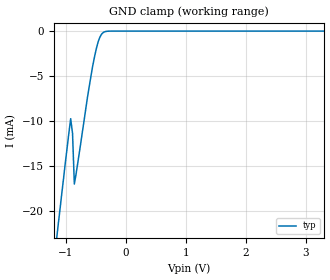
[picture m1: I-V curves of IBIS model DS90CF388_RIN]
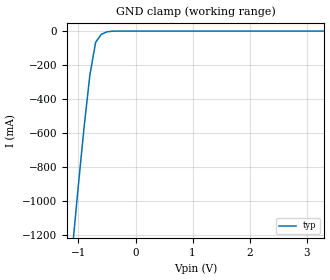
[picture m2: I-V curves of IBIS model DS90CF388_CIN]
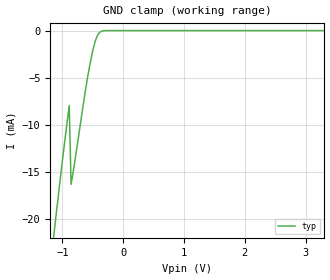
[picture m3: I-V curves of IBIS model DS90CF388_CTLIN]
|   National Semiconductor Corporation
|   Interface Products Group
|   IBIS Model of DS90CF388
|   100L TQFP Package
[IBIS Ver]   2.1
[File name]   90cf388.ibs
[File Rev]   1.0
[Date]   8/04/98
[Source]   File originated at National Semiconductor Corporation.
   Interface Group/Analog Division. All data based on
   measurements. CLKin and CLKout based on HSPICE sim.
[Notes]   File created/verfied by SBH.
[Disclaimer]
(C) Copyright National Semiconductor Corporation 1994
   All rights reserved
   National Semiconductor Corporation hereby grants
the user of this IBIS model a non-exclusive, nontransferable
license to use this IBIS model under the following terms.
Before using this IBIS model, the user should read this
license.  If the user does not accept these terms,  the
IBIS model should be returned to National within 30 days.
   The user is granted this license only to use the
IBIS model and is not granted rights to sell, load, rent,
lease or license the IBIS model in whole or in part, or in
modified form to anyone other than user. User may modify
the IBIS model to suit its specific applications but rights
to derivative works and such modifications shall belong to
National.
   This IBIS model is provided on an "AS IS" basis and
National makes absolutely no warranty with respect to the
information contained herein.NATIONAL DISCLAIMS AND CUSTOMER
WAIVES ALL WARRANTIES, EXPRESS OR IMPLIED, INCLUDING
WARRANTIES OF MERCHANTABILITY OR FITNESS FOR A PARTICULAR
PURPOSE. The entire risk as to quality and performance is
with the Customer. ACCORDINGLY, IN NO EVENT SHALL THE
COMPANY BE LIABLE FOR ANY DAMAGES, WHETHER IN CONTRACT OR
TORT,INCLUDING ANY LOST PROFITS OR OTHER INCIDENTAL,
CONSEQUENTIAL, EXEMPLARY, OR PUNITIVE DAMAGES ARISING OUT
OF THE USE OR APPLICATION OF THE IBIS model provided in
this package.Further, National reserves the right to make
changes without notice to any product herein to improve
reliability, function, or design. National does not convey
any license under patent rights or any other intellectual
property rights, including those of third parties.
   National is not obligated to provide maintenance or support
for the licensed IBIS model.
Contact National at ATTN:INTERFACE APPLICATIONS/IBIS MODELS.
2900 Semiconductor Drive, M/S A2595, Santa Clara, CA 95052-8090
[Copyright]   Copyright 1994, National Semiconductor, All Rights Reserved
[Component]   DS90CF388VJD
[Manufacturer]  National Semiconductor Corp
[Package]
|   typ   min   max
R_pkg   50.0m   NA   NA
L_pkg   2.52nH   NA   NA
C_pkg   0.11pF   NA   NA
[Pin]   signal_name  model_name   R_pin   L_pin   C_pin
1   PLLGND   GND   50.0m   2.40453n   0.17772p
2   PLLVCC   POWER   50.0m   2.2676n   0.1139p
3   PLLGND   GND   50.0m   2.28977n   0.10638p
4   DESKEW   DS90CF388_CTLIN   50.0m   2.30344n   0.10084p
5   PLLSEL   DS90CF388_CTLIN   50.0m   2.3344n   0.1p
6   BAL   DS90CF388_CTLIN   50.0m   2.35145n   0.1p
7   GND   GND   50.0m   2.41568n   0.1p
8   R10   DS90CF388_ROUT   50.0m   2.47482n   0.1p
9   R11   DS90CF388_ROUT   50.0m   2.5314n   0.1p
10   R12   DS90CF388_ROUT   50.0m   2.61993n   0.1p
11   R13   DS90CF388_ROUT   50.0m   2.69814n   0.1p
12   R14   DS90CF388_ROUT   50.0m   2.77365n   0.1p
13   VCC   POWER   50.0m   2.90748n   0.15p
14   R15   DS90CF388_ROUT   50.0m   2.91n   0.15p
15   R16   DS90CF388_ROUT   50.0m   2.78n   0.17p
16   GND   GND   50.0m   2.78n   0.17p
17   R17   DS90CF388_ROUT   50.0m   2.91n   0.15p
18   G10   DS90CF388_ROUT   50.0m   2.90748n   0.15p
19   G11   DS90CF388_ROUT   50.0m   2.77365n   0.1p
20   G12   DS90CF388_ROUT   50.0m   2.69814n   0.1p
21   G13   DS90CF388_ROUT   50.0m   2.61993n   0.1p
22   G14   DS90CF388_ROUT   50.0m   2.5314n   0.1p
23   VCC   POWER   50.0m   2.47482n   0.1p
24   G15   DS90CF388_ROUT   50.0m   2.41568n   0.1p
25   GND   GND   50.0m   2.35145n   0.1p
26   G16   DS90CF388_ROUT   50.0m   2.3344n   0.1p
27   G17   DS90CF388_ROUT   50.0m   2.30344n   0.10084p
28   B10   DS90CF388_ROUT   50.0m   2.28977n   0.10638p
29   B11   DS90CF388_ROUT   50.0m   2.2676n   0.1139p
30   B12   DS90CF388_ROUT   50.0m   2.40453n   0.17772p
31   B13   DS90CF388_ROUT   50.0m   2.40453n   0.17772p
32   B14   DS90CF388_ROUT   50.0m   2.2676n   0.1139p
33   VCC   POWER   50.0m   2.28977n   0.10638p
34   B15   DS90CF388_ROUT   50.0m   2.30344n   0.10084p
35   GND   GND   50.0m   2.3344n   0.1p
36   B16   DS90CF388_ROUT   50.0m   2.35145n   0.1p
37   B17   DS90CF388_ROUT   50.0m   2.41568n   0.1p
38   R20   DS90CF388_ROUT   50.0m   2.47482n   0.1p
39   R21   DS90CF388_ROUT   50.0m   2.5314n   0.1p
40   R22   DS90CF388_ROUT   50.0m   2.61993n   0.1p
41   R23   DS90CF388_ROUT   50.0m   2.69814n   0.1p
42   CLKOUT   DS90CF388_COUT   50.0m   2.77365n   0.1p
43   R24   DS90CF388_ROUT   50.0m   2.90748n   0.15p
44   GND   GND   50.0m   2.91n   0.15p
45   VCC   POWER   50.0m   2.78n   0.17p
46   R25   DS90CF388_ROUT   50.0m   2.78n   0.17p
47   R26   DS90CF388_ROUT   50.0m   2.91n   0.15p
48   R27   DS90CF388_ROUT   50.0m   2.90748n   0.15p
49   G20   DS90CF388_ROUT   50.0m   2.77365n   0.1p
50   G21   DS90CF388_ROUT   50.0m   2.69814n   0.1p
51   G22   DS90CF388_ROUT   50.0m   2.61993n   0.1p
52   G23   DS90CF388_ROUT   50.0m   2.5314n   0.1p
53   G24   DS90CF388_ROUT   50.0m   2.47482n   0.1p
54   GND   GND   50.0m   2.41568n   0.1p
55   G25   DS90CF388_ROUT   50.0m   2.35145n   0.1p
56   VCC   POWER   50.0m   2.3344n   0.1p
57   G26   DS90CF388_ROUT   50.0m   2.30344n   0.10084p
58   G27   DS90CF388_ROUT   50.0m   2.28977n   0.10638p
59   B20   DS90CF388_ROUT   50.0m   2.2676n   0.1139p
60   B21   DS90CF388_ROUT   50.0m   2.40453n   0.17772p
61   B22   DS90CF388_ROUT   50.0m   2.40453n   0.17772p
62   B23   DS90CF388_ROUT   50.0m   2.2676n   0.1139p
63   GND   GND   50.0m   2.28977n   0.10638p
64   B24   DS90CF388_ROUT   50.0m   2.30344n   0.10084p
65   B25   DS90CF388_ROUT   50.0m   2.3344n   0.1p
66   VCC   POWER   50.0m   2.35145n   0.1p
67   B26   DS90CF388_ROUT   50.0m   2.41568n   0.1p
68   B27   DS90CF388_ROUT   50.0m   2.47482n   0.1p
69   DE   DS90CF388_ROUT   50.0m   2.5314n   0.1p
70   VYSNC   DS90CF388_ROUT   50.0m   2.61993n   0.1p
71   HSYNC   DS90CF388_ROUT   50.0m   2.69814n   0.1p
72   GND   GND   50.0m   2.77365n   0.1p
73   STOPCLK   DS90CF388_ROUT   50.0m   2.90748n   0.15p
74   CNTLF/NC   NC   50.0m   2.91n   0.15p
75   CNTLE/NC   NC   50.0m   2.78n   0.17p
76   LVDSGND   GND   50.0m   2.78n   0.17p
77   R_FDE   DS90CF388_CTLIN   50.0m   2.91n   0.15p
78   PD   DS90CF388_CTLIN   50.0m   2.90748n   0.15p
79   A7P   DS90CF388_RIN   50.0m   2.77365n   0.1p
80   A7M   DS90CF388_RIN   50.0m   2.69814n   0.1p
81   LVDSVCC   POWER   50.0m   2.61993n   0.1p
82   A6P   DS90CF388_RIN   50.0m   2.5314n   0.1p
83   A6M   DS90CF388_RIN   50.0m   2.47482n   0.1p
84   A5P   DS90CF388_RIN   50.0m   2.41568n   0.1p
85   A5M   DS90CF388_RIN   50.0m   2.35145n   0.1p
86   A4P   DS90CF388_RIN   50.0m   2.3344n   0.1p
87   A4M   DS90CF388_RIN   50.0m   2.30344n   0.10084p
88   LVDSGND   GND   50.0m   2.28977n   0.10638p
89   A3P   DS90CF388_RIN   50.0m   2.2676n   0.1139p
90   A3M   DS90CF388_RIN   50.0m   2.40453n   0.17772p
91   CLKP   DS90CF388_CIN   50.0m   2.40453n   0.17772p
92   CLKM   DS90CF388_CIN   50.0m   2.2676n   0.1139p
93   LVDSVCC   POWER   50.0m   2.28977n   0.10638p
94   A2P   DS90CF388_RIN   50.0m   2.30344n   0.10084p
95   A2M   DS90CF388_RIN   50.0m   2.3344n   0.1p
96   A1P   DS90CF388_RIN   50.0m   2.35145n   0.1p
97   A1M   DS90CF388_RIN   50.0m   2.41568n   0.1p
98   A0P   DS90CF388_RIN   50.0m   2.47482n   0.1p
99   A0M   DS90CF388_RIN   50.0m   2.5314n   0.1p
100   LVDSGND   GND   50.0m   2.61993n   0.1p
[Diff_pin]   inv_pin   vdiff   tdelay_typ   tdelay_min   tdelay_max
| The '+' pin is Diff_pin and the '-' pin is the inv_pin
79   80   0.1   0   0   0
82   83   0.1   0   0   0
84   85   0.1   0   0   0
86   87   0.1   0   0   0
89   90   0.1   0   0   0
91   92   0.1   0   0   0
94   95   0.1   0   0   0
96   97   0.1   0   0   0
98   99   0.1   0   0   0
| Models and submodels in the file (5): DS90CF388_RIN (Input), DS90CF388_CIN (Input), DS90CF388_CTLIN (Input), DS90CF388_ROUT (Output), DS90CF388_COUT (Output)
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|   Receiver Input  MODEL
[Model]   DS90CF388_RIN
Model_type   Input
|Signals   A0P ~ A7P, A0M ~ A0M
Vinh = 2.0
Vinl = 0.8
|   typ   min   max
C_comp   5.070pF   NA   NA
|   typ   min   max
[Temperature Range]   25.0   -10   70
[Voltage range]   3.3V   3.0V   3.6V
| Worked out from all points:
|   GND clamp passes 1 mA (typ) near -0.45 V on its own axis
[Power_clamp]
| Note that the[POWER_clamp]voltage table is referenced to Vcc
| and is calculated using Vtable=Vcc - Vmeasured.
|Voltage   I(typ)   I(min)   I(max)
-3.3V     0A         0A         0A
3.3V      0A         0A         0A
[GND_clamp]
|Voltage   I(typ)   I(min)   I(max)
-3V       -130mA     NA         NA
-1.163V   -23.62mA   NA         NA
-1.133V   -21.82mA   NA         NA
-919mV    -9.711mA   NA         NA
-888mV    -11.34mA   NA         NA
-858mV    -16.96mA   NA         NA
-644mV    -7.566mA   NA         NA
-552mV    -3.872mA   NA         NA
-460mV    -1.169mA   NA         NA
-429mV    -625uA     NA         NA
-368mV    -119.5uA   NA         NA
3.3V      0A         NA         NA
|   Clock Input  MODEL
[Model]   DS90CF388_CIN
Model_type   Input
|Signals   CLKP, CLKM
Vinh = 2.0
Vinl = 0.8
|   typ   min   max
C_comp   5.070pF   NA   NA
|   typ   min   max
[Temperature Range]   25.0   -10   70
[Voltage range]   3.3V   3.0V   3.6V
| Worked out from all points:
|   GND clamp passes 1 mA (typ) near -0.41 V on its own axis
[Power_clamp]
| Note that the[POWER_clamp]voltage table is referenced to Vcc
| and is calculated using Vtable=Vcc - Vmeasured.
|Voltage   I(typ)   I(min)   I(max)
-3.3V     0A         0A         0A
3.3V      0A         0A         0A
[GND_clamp]
|Voltage   I(typ)   I(min)   I(max)
-3.3V     -9.725A    NA         NA
-1.1V     -1.256A    NA         NA
-1V       -899mA     NA         NA
-900mV    -559mA     NA         NA
-800mV    -258mA     NA         NA
-700mV    -66.1mA    NA         NA
-600mV    -19.3mA    NA         NA
-500mV    -4.31mA    NA         NA
-400mV    -468uA     NA         NA
3.3V      0A         NA         NA
|   Control  MODEL
[Model]   DS90CF388_CTLIN
Model_type   Input
|Signals   DESKEW,BAL,PLLSEL,R_FDE,PD*
Vinh = 2.0
Vinl = 0.8
|   typ   min   max
C_comp   5.429pF   NA   NA
|   typ   min   max
[Temperature Range]   25.0   -10   70
[Voltage range]   3.3V   3.0V   3.6V
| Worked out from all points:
|   GND clamp passes 1 mA (typ) near -0.45 V on its own axis
[GND_clamp]
|Voltage   I(typ)   I(min)   I(max)
-3V       -130mA     NA         NA
-1.133V   -21.26mA   NA         NA
-1.011V   -14.4mA    NA         NA
-888mV    -7.957mA   NA         NA
-858mV    -16.34mA   NA         NA
-797mV    -13.94mA   NA         NA
-613mV    -6.037mA   NA         NA
-521mV    -2.717mA   NA         NA
-460mV    -1.117mA   NA         NA
-429mV    -589.7uA   NA         NA
-368mV    -100.1uA   NA         NA
3.3V      0A         NA         NA
[Power_clamp]
| Note that the[POWER_clamp]voltage table is referenced to Vcc
| and is calculated using Vtable=Vcc - Vmeasured.
|Voltage   I(typ)   I(min)   I(max)
-3.3V     0A         0A         0A
3.3V      0A         0A         0A
